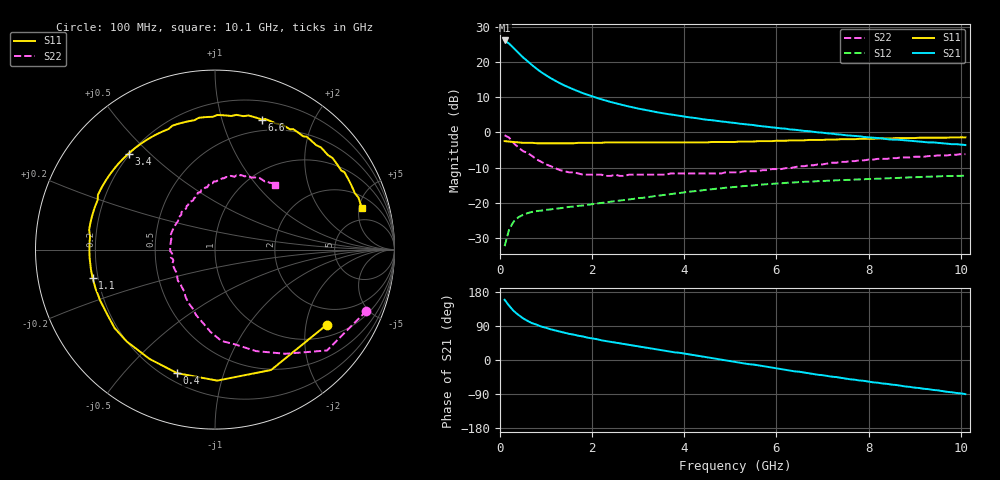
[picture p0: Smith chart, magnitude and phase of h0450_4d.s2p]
!HBFP-0450
!S and NOISE PARAMETERS at Vce=4V  Ic=10mA.  LAST UPDATED  09-04-98
# GHZ S MA R  50
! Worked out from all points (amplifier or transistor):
!   101 points, 100 MHz to 10.1 GHz, reference 50 ohm
!   highest |S21| = 26.2 dB at 100 MHz (marker M1)
!   |S21| within 3 dB of that: start of sweep to 360.4 MHz
!   unconditionally stable (mu >= 1): 2.729 GHz to end of sweep
!   at 1.7 GHz: K = 0.75, MSG = 16.3 dB, |S12| = -20.9 dB
!   at 5.1 GHz: K = 1.17, MAG = 6.6 dB, |S12| = -15.5 dB
!   at 10.1 GHz: K = 1.07, MAG = 2.7 dB, |S12| = -12.3 dB
!   lowest NFmin = 1.19 dB at 1.8 GHz
!   S11 on the Smith chart (normalised r, x): 100 MHz: 1.37, -2.63; 400 MHz: 0.25, -0.71; 1.1 GHz: 0.18, -0.11; 3.4 GHz: 0.19, +0.43; 6.6 GHz: 0.38, +1.36; 10.1 GHz: 3.14, +5.30
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0.1  0.75 -34.0  20.34 159.0  0.024 68.0  0.91 -22.0
0.2  0.74 -65.0  18.27 143.0  0.042 55.0  0.84 -42.0
0.3  0.73 -89.0  15.78 129.0  0.054 47.0  0.7 -56.0
0.4  0.72 -107.0  13.56 119.0  0.062 41.0  0.61 -68.0
0.5  0.71 -121.0  11.68 110.0  0.067 36.0  0.54 -78.0
0.6  0.71 -134.0  10.29 103.0  0.071 32.0  0.51 -86.0
0.7  0.71 -142.0  9.02 97.0  0.074 29.0  0.46 -93.0
0.8  0.7 -150.0  7.99 93.0  0.076 27.0  0.41 -100.0
0.9  0.7 -156.0  7.16 88.0  0.077 26.0  0.38 -106.0
1.1  0.7 -167.0  5.91 81.0  0.08 24.0  0.33 -117.0
1.4  0.7 -179.0  4.65 72.0  0.085 23.0  0.28 -131.0
1.8  0.71 168.0  3.61 62.0  0.091 22.0  0.25 -148.0
2.2  0.71 157.0  2.96 52.0  0.099 21.0  0.25 -162.0
2.4  0.72 152.0  2.71 48.0  0.103 21.0  0.24 -167.0
2.8  0.72 144.0  2.33 40.0  0.111 19.0  0.25 -178.0
3.4  0.72 132.0  1.94 28.0  0.125 16.0  0.25 169.0
3.5  0.72 130.0  1.89 26.0  0.127 15.0  0.25 167.0
5.1  0.73 99.0  1.36 -5.0  0.167 0.0  0.27 136.0
6.6  0.77 70.0  1.05 -33.0  0.198 -19.0  0.33 104.0
6.8  0.78 67.0  1.02 -37.0  0.2 -21.0  0.34 101.0
8.5  0.82 40.0  0.79 -65.0  0.223 -42.0  0.43 74.0
10.1  0.85 16.0  0.66 -90.0  0.242 -64.0  0.49 47.0
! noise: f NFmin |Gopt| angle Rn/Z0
1.8  1.19  0.46  -179  0.05
2  1.22  0.48  -175  0.05
2.5  1.39  0.52  -161  0.07
3.5  1.68  0.61  -138  0.15
4  1.91  0.63  -125  0.26
5  2.21  0.67  -103  0.57
5.5  2.39  0.71  -92  0.83
7  2.87  0.76  -63  1.96
8  3.24  0.79  -46  3
10  3.84  0.82  -16  5.22
